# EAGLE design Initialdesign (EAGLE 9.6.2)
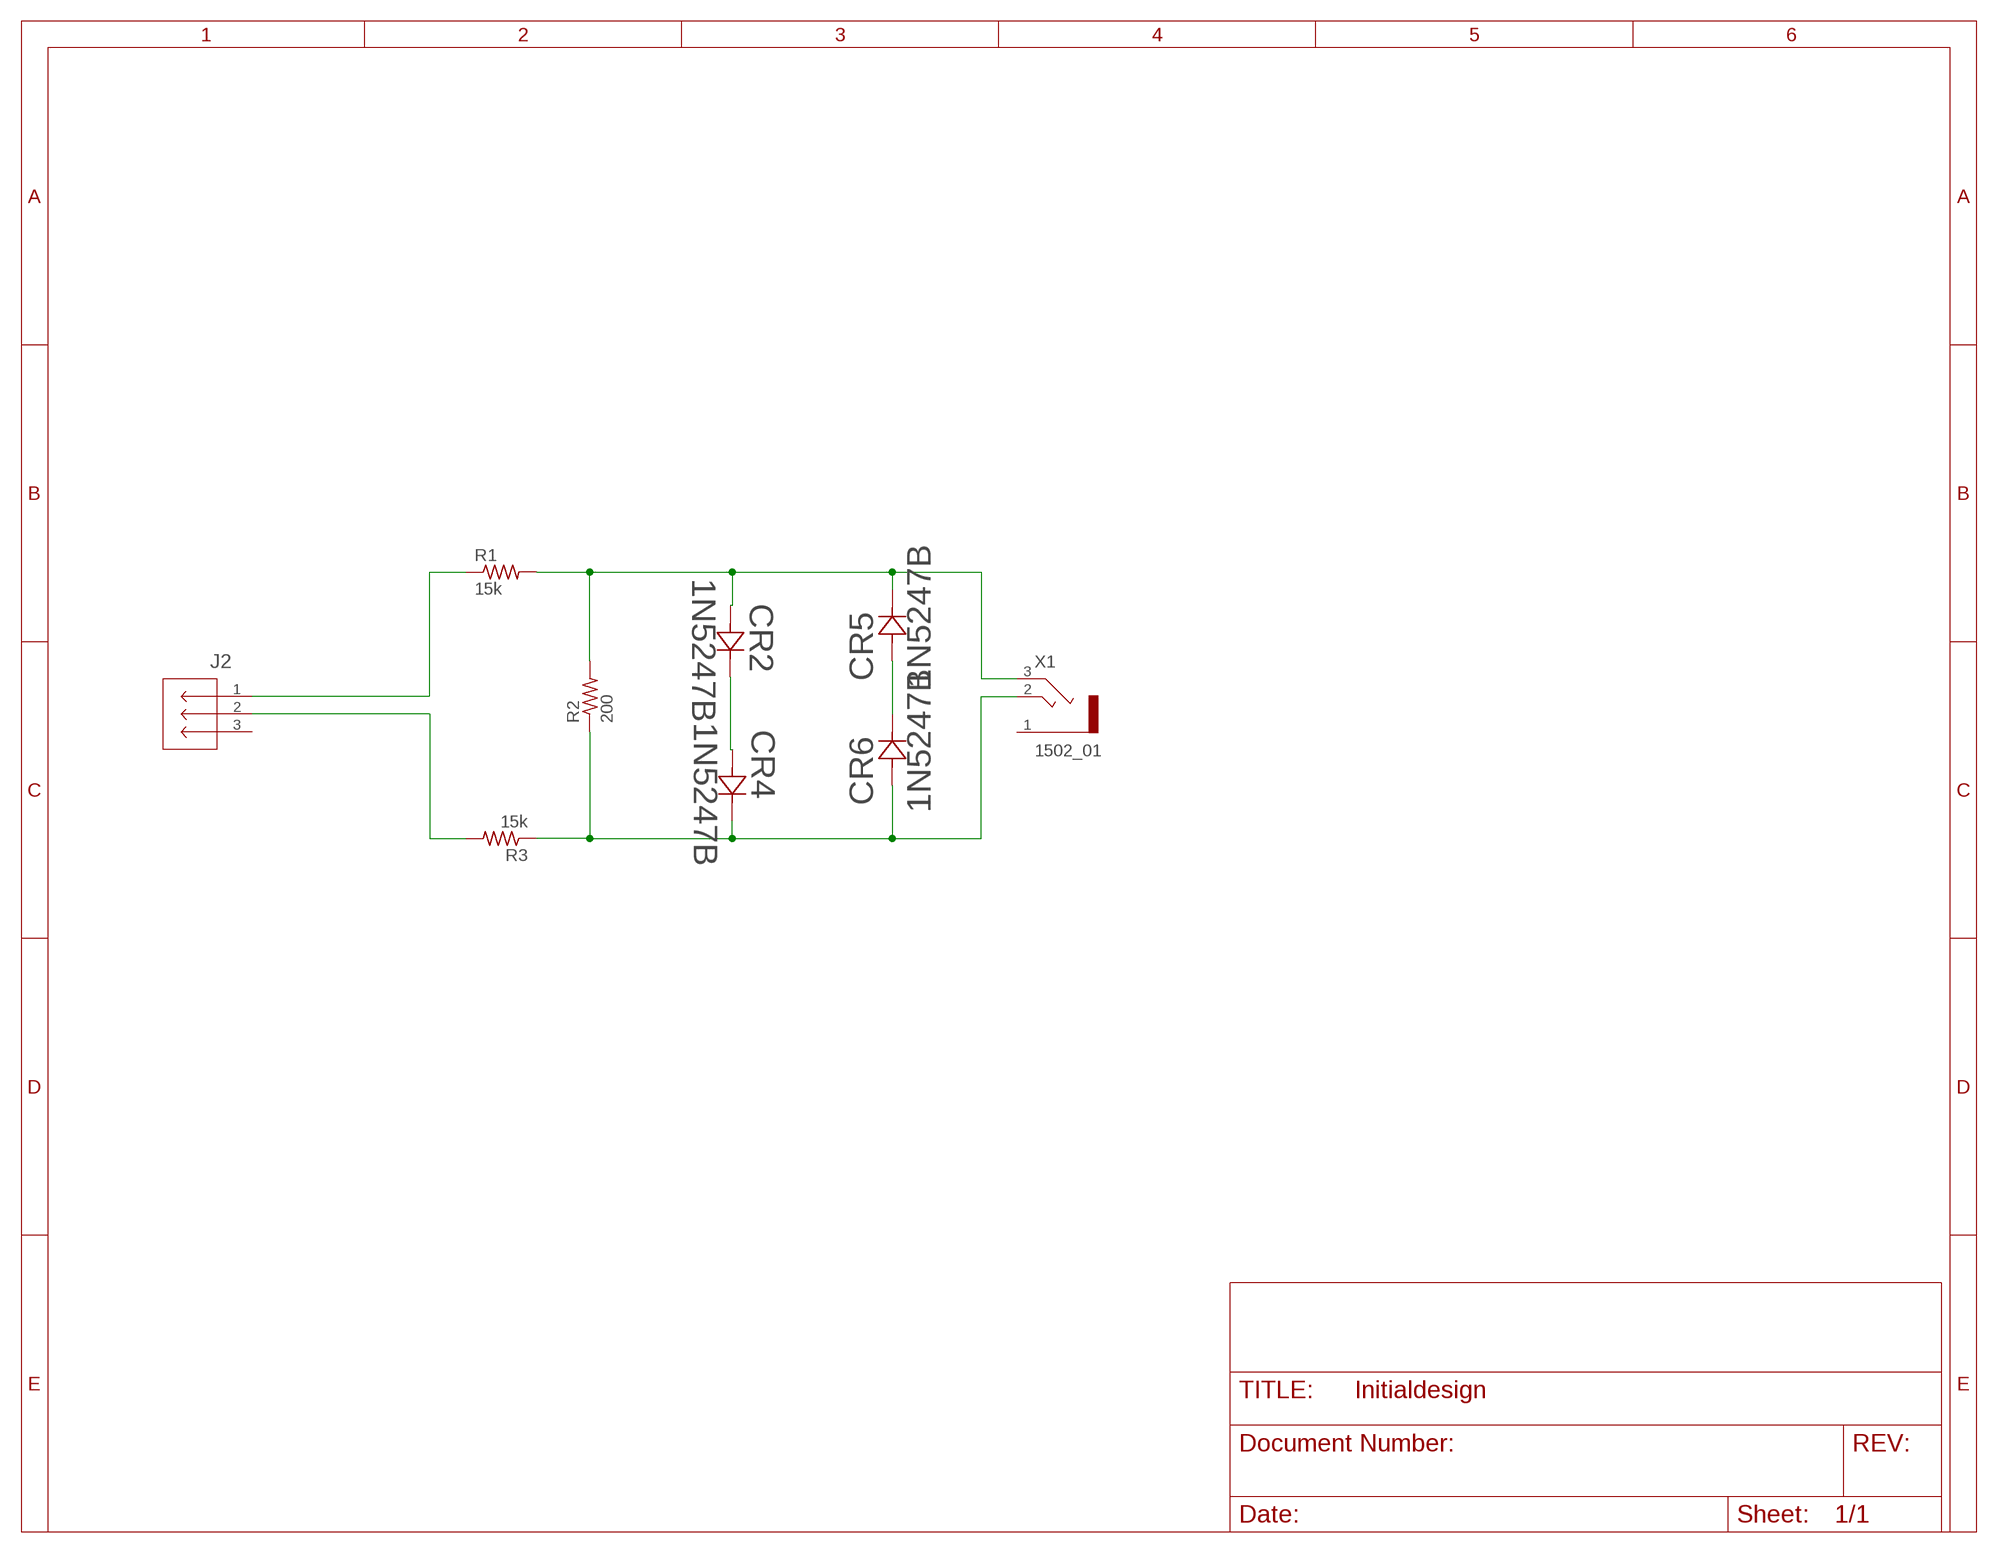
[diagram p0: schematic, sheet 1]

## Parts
CR2  1N5247B  [AFL-W2C8.9D]
CR4  1N5247B  [AFL-W2C8.9D]
CR5  1N5247B  [AFL-W2C8.9D]
CR6  1N5247B  [AFL-W2C8.9D]
J2  282841-3  [CONN3_282841-3_TEC]
R1  15k  R-US_0204/7  [0204/7]
R2  200  R-US_0204/7  [0204/7]
R3  15k  R-US_0204/7  [0204/7]
X1  1502_01  [1502_01]

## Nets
N$1: CR2.1 CR4.2
N$2: CR2.2 CR5.1 R1.2 R2.2 X1.3
N$3: CR5.2 CR6.1
N$5: J2.1 R1.1
N$6: J2.2 R3.2
N$7: CR4.1 CR6.2 R2.1 R3.1 X1.2
Unconnected: J2.3 X1.1

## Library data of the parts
CR2 CR4-CR6 = 1N5257B:1N5247B; COPYRIGHT: Copyright (C) 2022 Ultra Librarian. All rights reserved.; MANUFACTURER_PART_NUMBER: 1N5247B; MFR_NAME: onsemi
J2 = 282841-3:282841-3; COPYRIGHT: Copyright (C) 2022 Ultra Librarian. All rights reserved.; MANUFACTURER_PART_NUMBER: 282841-3; MFR_NAME: TE Connectivity
R1-R3 = rcl:R-US_: RESISTOR, American symbol; SPICEPREFIX: R
X1 = con-lumberg:1502_01: Jack connectors according to JISC 6560, 3.5 mm Klinkensteckverbinder nach JISC 6560, 3,5 mm Source: http://www.lumberg.com/Produkte/PDFs/1502_01.pdf; OC_FARNELL: 4739747; OC_NEWARK: unknown

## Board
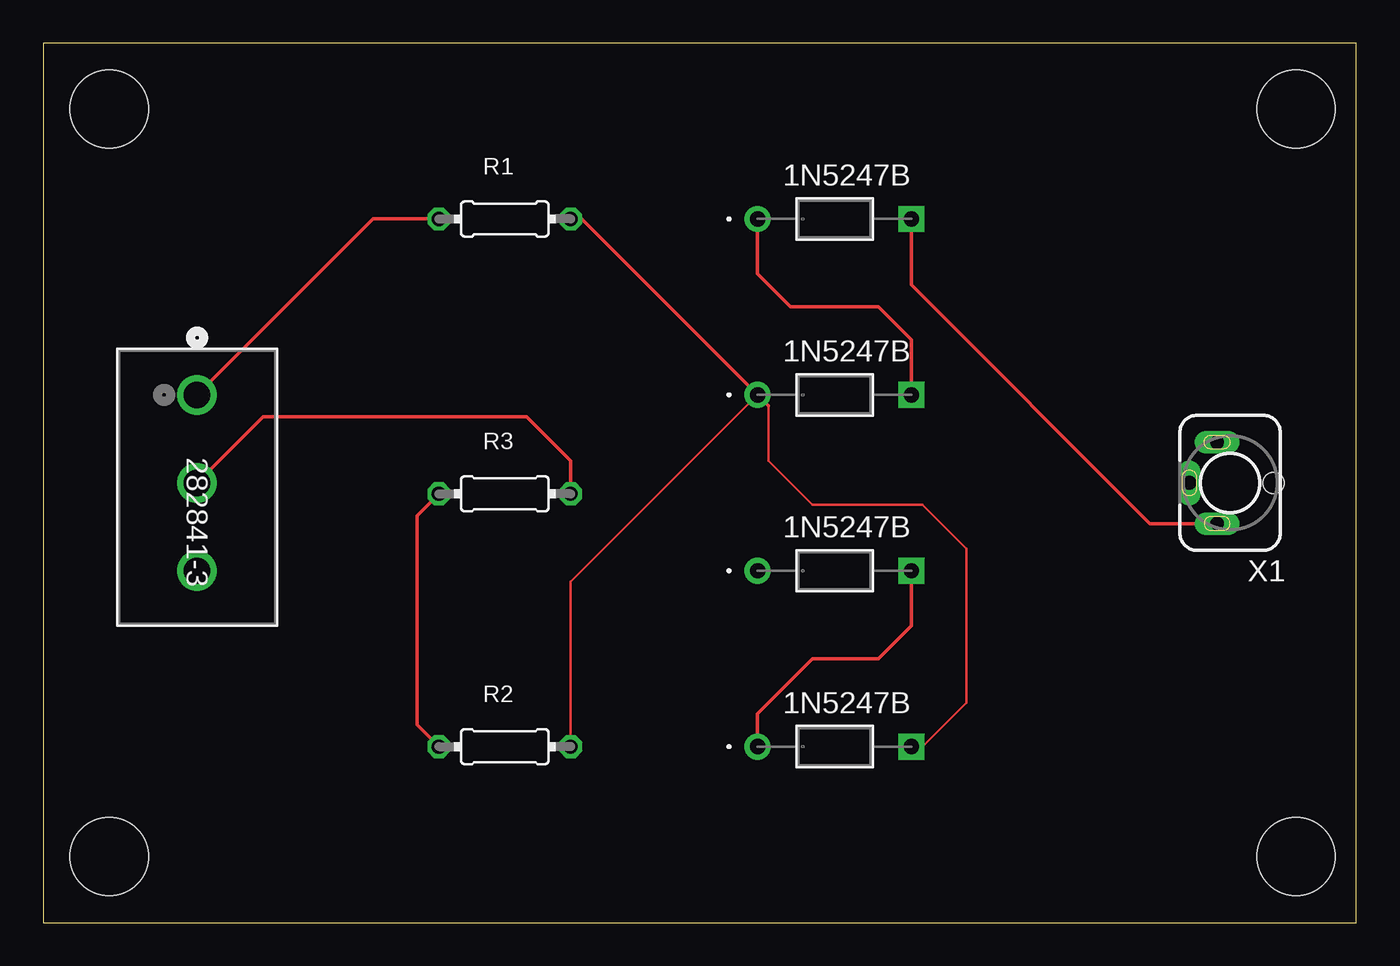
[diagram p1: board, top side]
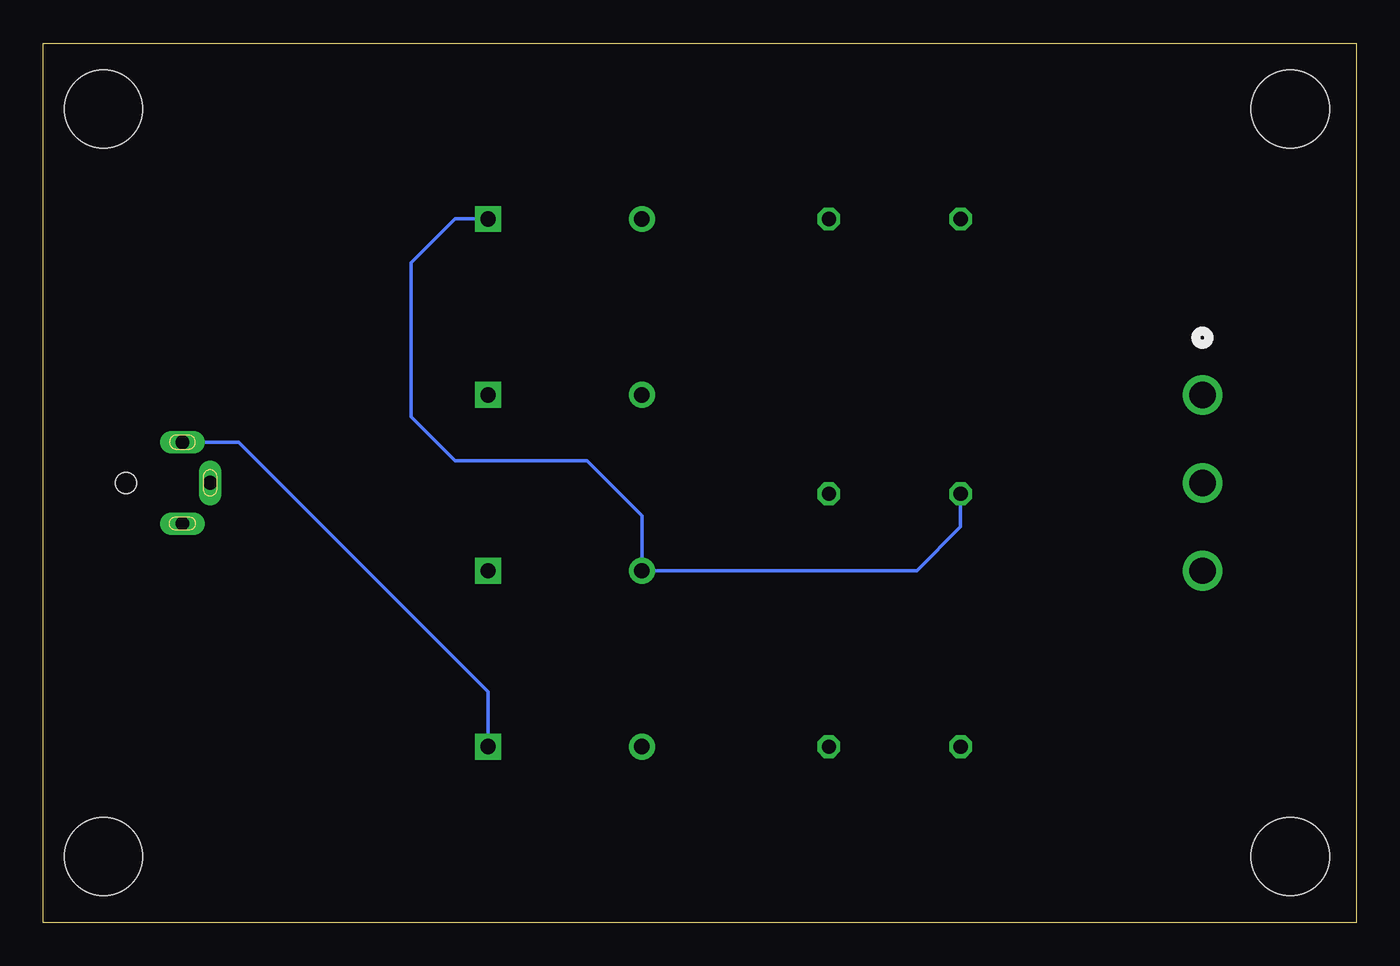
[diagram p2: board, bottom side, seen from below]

Size 75.87 x 50.79 mm. Coordinates in mm from the lower left corner, seen from the top.
Outline: 0,0 75.87,0 75.87,50.79 0,50.79 0,0
Copper layers (1*16): Top 0.035mm / dielectric 1.5mm / Bottom 0.035mm
Design rules "default": minimum track width 6mil, minimum drill 0.35mm, track to track 6mil, track to pad 6mil, pad to pad 6mil, via to via 6mil, smd to smd 6mil, copper to edge 40mil, drill to drill 6mil, minimum pad ring 10mil, minimum via ring 8mil, stop-mask expansion 4mil, vias tented up to drill 0mil, thermal gap 10mil
Holes 4.5 mm at 3.81,46.99 3.81,3.81 72.39,3.81 72.39,46.99

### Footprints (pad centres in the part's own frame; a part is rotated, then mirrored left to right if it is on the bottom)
AFL-W2C8.9D = drill 0.889 pad 1.499: 1 -8.89,0 | drill 0.889 pad 1.499 square: 2 0,0
CONN3_282841-3_TEC = drill 1.524 pad 2.032: 1 0,0; 2 5.08,0; 3 10.16,0
0204/7 = drill 0.813 octagon: 1 -3.81,0; 2 3.81,0
1502_01 = drill 0.8 pad 1.2 long: 1 0,2.35; 2 -2.35,0.75; 3 2.35,0.75 | hole 1.2: 0,-2.5

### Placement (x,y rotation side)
CR2  50.16,10.16 0 top
CR4  50.16,20.32 0 top
CR5  50.16,30.48 0 top
CR6  50.16,40.64 0 top
J2  8.89,30.48 270 top
R1  26.67,40.64 0 top
R2  26.67,10.16 0 top
R3  26.67,24.77 0 top
X1  68.58,25.4 90 top

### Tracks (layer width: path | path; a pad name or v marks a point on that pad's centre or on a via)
N$1
  Top 0.203: CR4.2 50.16,17.14 48.26,15.24 44.45,15.24 41.27,12.06 CR2.1
N$2
  Top 0.152: CR5.1 30.48,19.68 R2.2 | 41.91,29.84 41.91,26.67 44.45,24.13 50.8,24.13 53.34,21.59 53.34,12.7 50.8,10.16
  Top 0.203: R1.2 31.11,40.64 CR5.1 41.91,29.84 | 50.8,10.16 CR2.2
  Bottom 0.203: CR2.2 50.16,13.34 64.58,27.75 X1.3
N$3
  Top 0.203: CR6.1 41.27,37.47 43.18,35.56 48.26,35.56 50.16,33.66 CR5.2
N$5
  Top 0.203: R1.1 19.05,40.64 J2.1
N$6
  Top 0.203: R3.2 30.48,26.67 27.94,29.21 12.7,29.21 J2.2
N$7
  Top 0.203: R3.1 21.59,23.5 21.59,11.43 R2.1 | CR6.2 50.16,36.83 63.95,23.05 X1.2
  Bottom 0.203: R3.1 22.86,22.86 25.4,20.32 CR4.1 41.27,23.5 44.45,26.67 52.07,26.67 54.61,29.21 54.61,38.1 52.07,40.64 CR6.2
